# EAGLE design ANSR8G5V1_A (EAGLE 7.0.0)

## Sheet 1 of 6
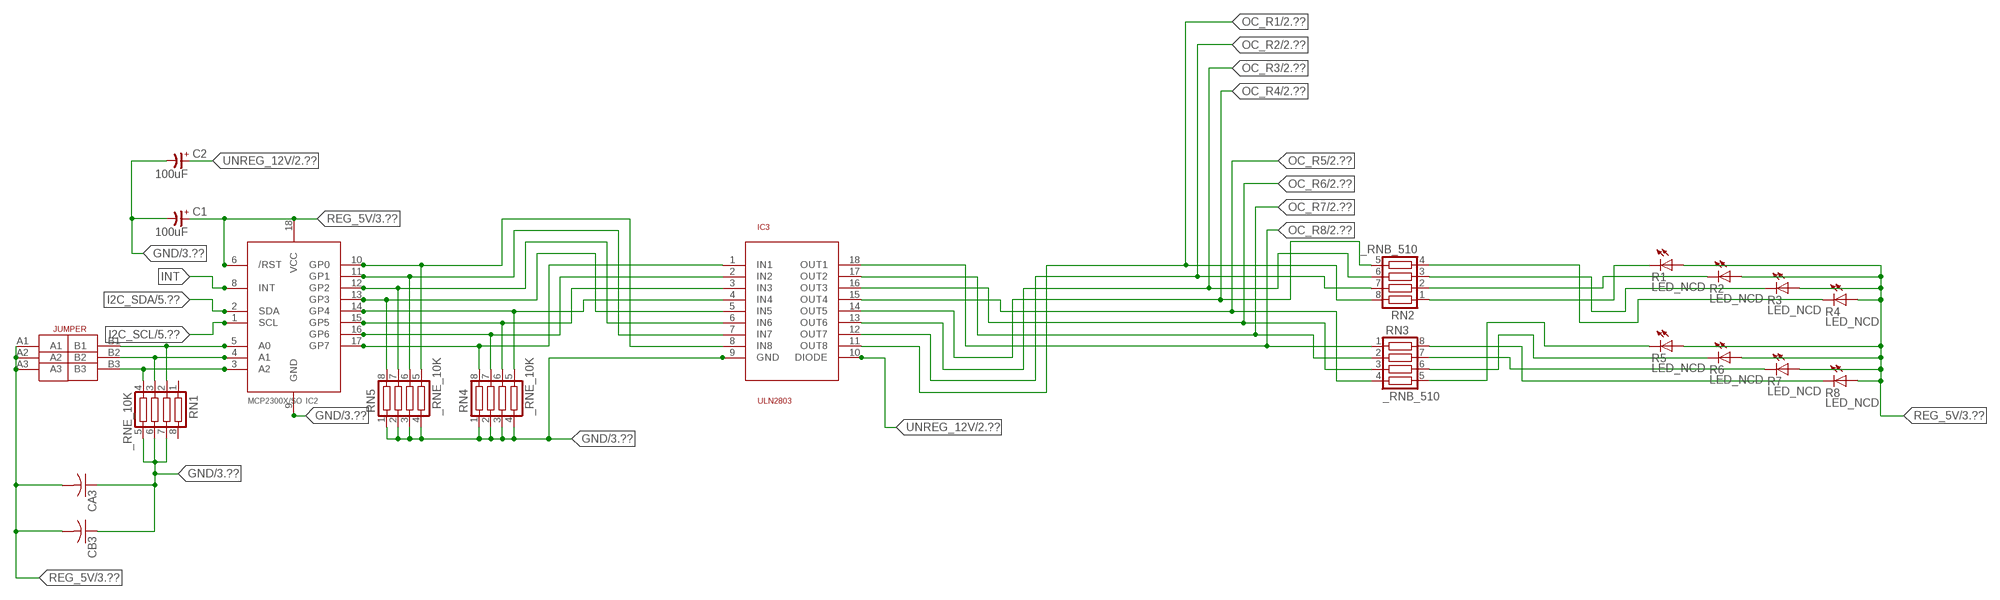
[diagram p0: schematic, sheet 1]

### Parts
C1  100uF  CP-E-025X060  [E-025X060]
C2  100uF  CP-E-025X060  [E-025X060]
CA3  CC1206KRX7R9BB104C1206K  [CC1206KRX7R9BB104]
CB3  TMK316F106ZL-TC1206K  [TMK316F106ZL-T]
IC2  MCP2300X/SO  [SO18W]
IC3  ULN2803  [SO18L]
R1  LED_NCD  [CHIPLED_0603]
R2  LED_NCD  [CHIPLED_0603]
R3  LED_NCD  [CHIPLED_0603]
R4  LED_NCD  [CHIPLED_0603]
R5  LED_NCD  [CHIPLED_0603]
R6  LED_NCD  [CHIPLED_0603]
R7  LED_NCD  [CHIPLED_0603]
R8  LED_NCD  [CHIPLED_0603]
RN1  _RNE_10K  [RNE]
RN2  _RNB_510  [RNB]
RN3  _RNB_510  [RNB]
RN4  _RNE_10K  [RNE]
RN5  _RNE_10K  [RNE]
U$18  JUMPER_3X2  [JUMPER_3X2]

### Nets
GND: C1.- C2.- CA3.1 CB3.1 IC2.9(GND) IC3.9(GND) RN1.5 RN1.6 RN1.7 RN4.1 RN4.2 RN4.3 RN4.4 RN5.1 RN5.2 RN5.3 RN5.4 ; also sheet 3,4,5,6
GP4: IC2.14(GP4) IC3.4(IN4) RN4.5
GP6: IC2.16(GP6) IC3.2(IN2) RN4.7
I2C_SCL: IC2.1(SCL) ; also sheet 5,6
I2C_SDA: IC2.2(SDA) ; also sheet 5,6
INT: IC2.8(INT)
N$6: IC2.5(A0) RN1.2 U$18.B1
N$7: IC2.4(A1) RN1.3 U$18.B2
N$8: IC2.3(A2) RN1.4 U$18.B3
N$20: R1.C RN2.1
N$21: IC2.12(GP2) IC3.6(IN6) RN5.7
N$22: IC2.11(GP1) IC3.7(IN7) RN5.6
N$23: IC2.10(GP0) IC3.8(IN8) RN5.5
N$29: R2.C RN2.2
N$30: R3.C RN2.3
N$31: R4.C RN2.4
N$32: R8.C RN3.8
N$81: R7.C RN3.7
N$82: R6.C RN3.6
N$83: R5.C RN3.5
N$89: IC2.13(GP3) IC3.5(IN5) RN5.8
N$93: IC2.15(GP5) IC3.3(IN3) RN4.6
N$94: IC2.17(GP7) IC3.1(IN1) RN4.8
OC_R1: IC3.11(OUT8) RN2.8 ; also sheet 2
OC_R2: IC3.12(OUT7) RN2.7 ; also sheet 2
OC_R3: IC3.13(OUT6) RN2.6 ; also sheet 2
OC_R4: IC3.14(OUT5) RN2.5 ; also sheet 2
OC_R5: IC3.15(OUT4) RN3.4 ; also sheet 2
OC_R6: IC3.16(OUT3) RN3.3 ; also sheet 2
OC_R7: IC3.17(OUT2) RN3.2 ; also sheet 2
OC_R8: IC3.18(OUT1) RN3.1 ; also sheet 2
REG_5V: C1.+ CA3.2 CB3.2 IC2.6(/RST) IC2.18(VCC) R1.A R2.A R3.A R4.A R5.A R6.A R7.A R8.A U$18.A1 U$18.A2 U$18.A3 ; also sheet 3,4,5,6
UNREG_12V: C2.+ IC3.10(DIODE) ; also sheet 2,3
Unconnected: RN1.1 RN1.8

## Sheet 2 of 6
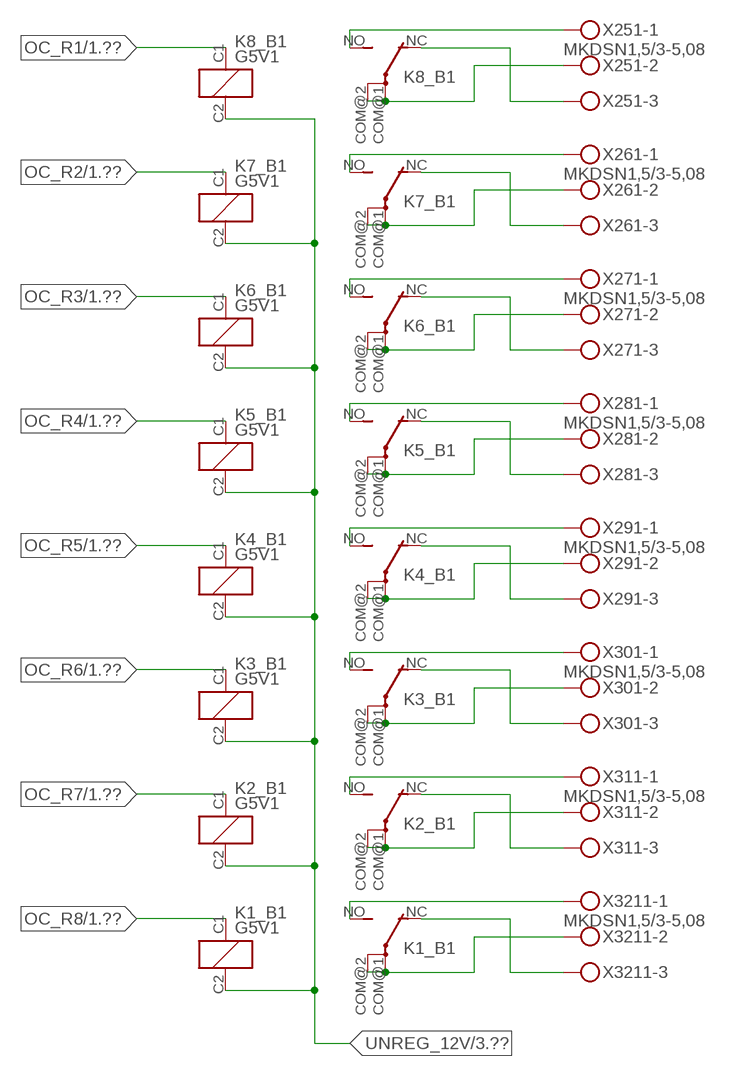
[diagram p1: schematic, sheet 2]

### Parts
K1_B1  G5V1  [G5V1]
K2_B1  G5V1  [G5V1]
K3_B1  G5V1  [G5V1]
K4_B1  G5V1  [G5V1]
K5_B1  G5V1  [G5V1]
K6_B1  G5V1  [G5V1]
K7_B1  G5V1  [G5V1]
K8_B1  G5V1  [G5V1]
X251  MKDSN1,5/3-5,08  [MKDSN1,5/3-5,08]
X261  MKDSN1,5/3-5,08  [MKDSN1,5/3-5,08]
X271  MKDSN1,5/3-5,08  [MKDSN1,5/3-5,08]
X281  MKDSN1,5/3-5,08  [MKDSN1,5/3-5,08]
X291  MKDSN1,5/3-5,08  [MKDSN1,5/3-5,08]
X301  MKDSN1,5/3-5,08  [MKDSN1,5/3-5,08]
X311  MKDSN1,5/3-5,08  [MKDSN1,5/3-5,08]
X3211  MKDSN1,5/3-5,08  [MKDSN1,5/3-5,08]

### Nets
N$203: K8_B1.COM@1(2:P) K8_B1.COM@2(2:P) X251.2
N$204: K8_B1.NC(2:O) X251.3
N$205: K8_B1.NO(2:S) X251.1
N$206: K7_B1.NO(2:S) X261.1
N$207: K6_B1.NO(2:S) X271.1
N$208: K7_B1.NC(2:O) X261.3
N$209: K7_B1.COM@1(2:P) K7_B1.COM@2(2:P) X261.2
N$210: K6_B1.NC(2:O) X271.3
N$211: K6_B1.COM@1(2:P) K6_B1.COM@2(2:P) X271.2
N$212: K5_B1.NC(2:O) X281.3
N$213: K5_B1.COM@1(2:P) K5_B1.COM@2(2:P) X281.2
N$214: K5_B1.NO(2:S) X281.1
N$215: K4_B1.NO(2:S) X291.1
N$216: K4_B1.NC(2:O) X291.3
N$217: K4_B1.COM@1(2:P) K4_B1.COM@2(2:P) X291.2
N$218: K3_B1.NO(2:S) X301.1
N$219: K3_B1.NC(2:O) X301.3
N$220: K3_B1.COM@1(2:P) K3_B1.COM@2(2:P) X301.2
N$221: K2_B1.NO(2:S) X311.1
N$222: K2_B1.NC(2:O) X311.3
N$223: K2_B1.COM@1(2:P) K2_B1.COM@2(2:P) X311.2
N$224: K1_B1.NO(2:S) X3211.1
N$225: K1_B1.NC(2:O) X3211.3
N$226: K1_B1.COM@1(2:P) K1_B1.COM@2(2:P) X3211.2
OC_R1: K8_B1.C1(1:C1) ; also sheet 1
OC_R2: K7_B1.C1(1:C1) ; also sheet 1
OC_R3: K6_B1.C1(1:C1) ; also sheet 1
OC_R4: K5_B1.C1(1:C1) ; also sheet 1
OC_R5: K4_B1.C1(1:C1) ; also sheet 1
OC_R6: K3_B1.C1(1:C1) ; also sheet 1
OC_R7: K2_B1.C1(1:C1) ; also sheet 1
OC_R8: K1_B1.C1(1:C1) ; also sheet 1
UNREG_12V: K1_B1.C2(1:C2) K2_B1.C2(1:C2) K3_B1.C2(1:C2) K4_B1.C2(1:C2) K5_B1.C2(1:C2) K6_B1.C2(1:C2) K7_B1.C2(1:C2) K8_B1.C2(1:C2) ; also sheet 1,3

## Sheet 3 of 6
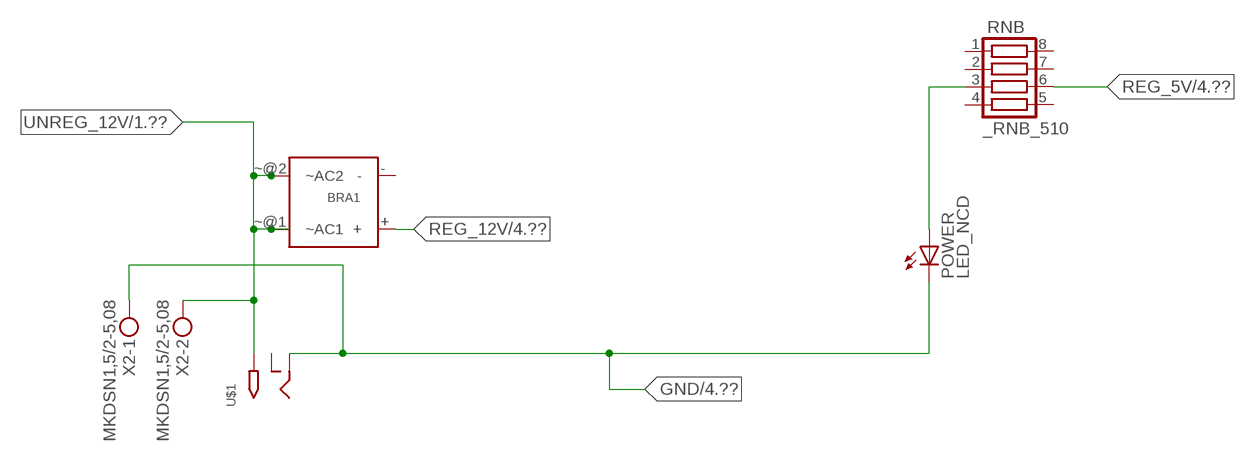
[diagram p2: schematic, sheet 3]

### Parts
BRA1  MB2S_  [MB2S]
POWER  LED_NCD  [CHIPLED_0603]
RNB  _RNB_510  [RNB]
U$1  2.1MMJACK  [PJ-102A]
X2  MKDSN1,5/2-5,08  [MKDSN1,5/2-5,08]

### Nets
GND: POWER.C U$1.RING X2.1 ; also sheet 1,4,5,6
N$2: POWER.A RNB.3
REG_5V: RNB.6 ; also sheet 1,4,5,6
REG_12V: BRA1.+ ; also sheet 4
UNREG_12V: BRA1.~@1(~AC1) BRA1.~@2(~AC2) U$1.TIP X2.2 ; also sheet 1,2
Unconnected: BRA1.- RNB.1 RNB.2 RNB.4 RNB.5 RNB.7 RNB.8 U$1.RING_SW

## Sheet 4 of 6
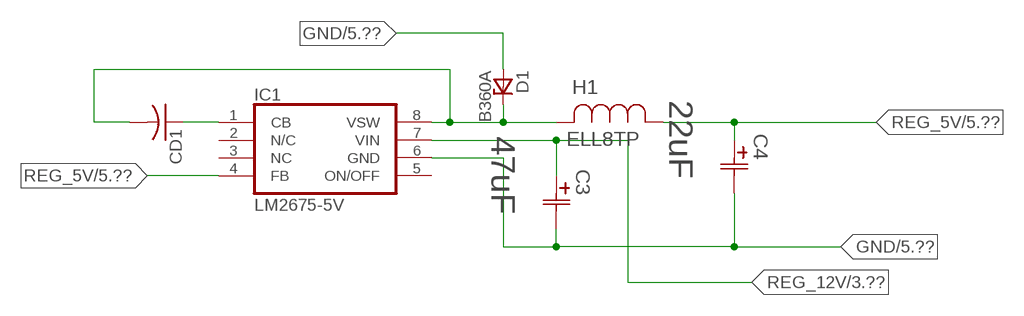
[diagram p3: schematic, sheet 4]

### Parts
C3  47uF  490-5463-6-NDCAP  [C2917(7343)-Y]
C4  22uF  490-5463-6-NDCAP  [C2917(7343)-Y]
CD1  _CD_10NF_50VC1206K  [_CD_10NF_50V]
D1  B360A  [DO214AC_ZENER]
H1  ELL8TP  [IND_ELL8TP]
IC1  LM2675-5V  LM2675  [SO-8]

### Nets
GND: C3.2(C2) C4.2(C2) D1.A IC1.6(GND) ; also sheet 1,3,5,6
N$1: CD1.2 D1.C H1.2 IC1.8(VSW)
N$3: CD1.1 IC1.1(CB)
REG_5V: C4.1(C1) H1.1 IC1.4(FB) ; also sheet 1,3,5,6
REG_12V: C3.1(C1) IC1.7(VIN) ; also sheet 3
Unconnected: IC1.2(N/C) IC1.5(ON/OFF)

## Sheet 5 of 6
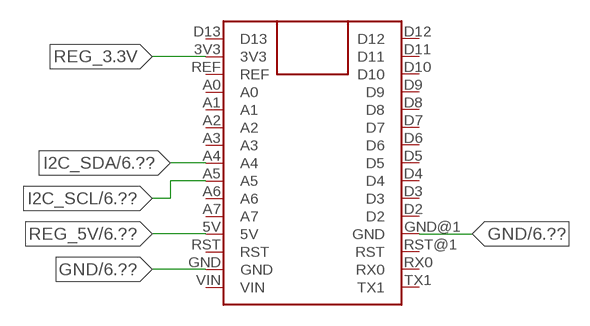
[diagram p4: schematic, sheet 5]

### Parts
FOR_NANO  ARDUINO_NANO  [ARDUINO_NANO]

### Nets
GND: FOR_NANO.GND FOR_NANO.GND@1(GND) ; also sheet 1,3,4,6
I2C_SCL: FOR_NANO.A5 ; also sheet 1,6
I2C_SDA: FOR_NANO.A4 ; also sheet 1,6
REG_3.3V: FOR_NANO.3V3
REG_5V: FOR_NANO.5V ; also sheet 1,3,4,6
Unconnected: FOR_NANO.A0 FOR_NANO.A1 FOR_NANO.A2 FOR_NANO.A3 FOR_NANO.A6 FOR_NANO.A7 FOR_NANO.D2 FOR_NANO.D3 FOR_NANO.D4 FOR_NANO.D5 FOR_NANO.D6 FOR_NANO.D7 FOR_NANO.D8 FOR_NANO.D9 FOR_NANO.D10 FOR_NANO.D11 FOR_NANO.D12 FOR_NANO.D13 FOR_NANO.REF FOR_NANO.RST FOR_NANO.RST@1(RST) FOR_NANO.RX0 FOR_NANO.TX1 FOR_NANO.VIN

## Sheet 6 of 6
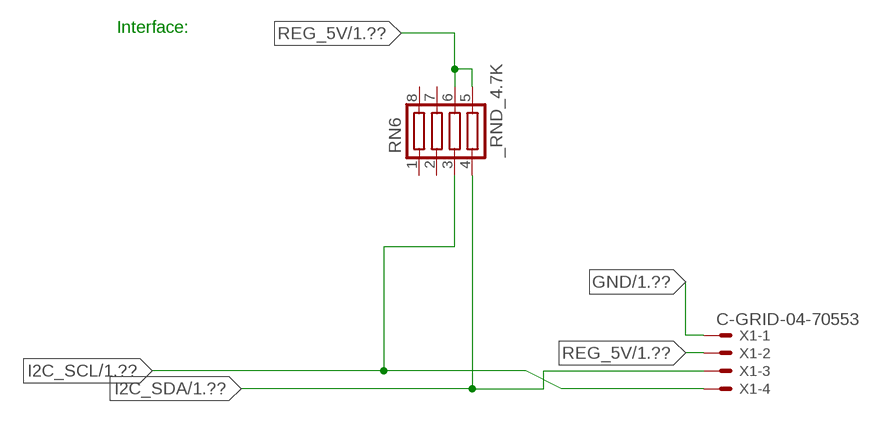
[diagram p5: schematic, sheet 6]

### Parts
RN6  _RND_4.7K  [RND]
X1  C-GRID-04-70553  [70553-04]

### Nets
GND: X1.1 ; also sheet 1,3,4,5
I2C_SCL: RN6.3 X1.4 ; also sheet 1,5
I2C_SDA: RN6.4 X1.3 ; also sheet 1,5
REG_5V: RN6.5 RN6.6 X1.2 ; also sheet 1,3,4,5
Unconnected: RN6.1 RN6.2 RN6.7 RN6.8

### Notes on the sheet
- Interface:

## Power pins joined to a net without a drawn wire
NC: IC1.3(NC)

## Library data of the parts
BRA1 = NCD_ULTIMATE_LIBRARY:MB2S: Bridge Rectifier BRA MB2S 200V 500ma Digikey MB2S-TPMSTR-ND/MB2S-TP
C1 C2 = NCD_ULTIMATE_LIBRARY:CP-: Capacitors All Kinds POLARIZED CAP
C3 C4 = NCD_ULTIMATE_bhaskar:490-5463-6-ND: NCD CAP
CA3 = NCD_ULTIMATE_LIBRARY:CC1206KRX7R9BB104: Capacitor CA .1uF 50V SMT C1206K CC1206KRX7R9BB104
CB3 = NCD_ULTIMATE_LIBRARY:TMK316F106ZL-T: Capacitor CB 10uF SMT 1206 TMK316F106ZL-T
CD1 = NCD_ULTIMATE_LIBRARY:_CD_10NF_50V: Capacitor 10nF SMT
D1 = NCD_ULTIMATE_bhaskar:B360A: NCD DIODE B350A/B360A
FOR_NANO = NCD_ULTIMATE_CONNECTORS:ARDUINO_NANO
H1 = NCD_ULTIMATE_bhaskar:ELL8TP: NCD coil
IC1 = NCD_ULTIMATE_bhaskar:LM2675: LM2675 NCD http://www.ti.com/lit/ds/symlink/lm2675.pdf
IC2 = NCD_ULTIMATE_LIBRARY:MCP2300X: Semiconductor Port Expander I/O 8-Bit I2C MCP23008 Inexpensive i2c i/o expander - 8 general purpose i/o pins with optional pullups
IC3 = NCD_ULTIMATE_LIBRARY:ULN2803: Semiconductor 8 O.C. N-Channel Transistor Driver Digikey ULN2803AFWGCELTR-ND/ULN2803AFWG,C,EL
K1_B1 K2_B1 K3_B1 K4_B1 K5_B1 K6_B1 K7_B1 K8_B1 = NCD_ULTIMATE_LIBRARY:G5V1: RELAY 1 x switch, 0.5 A/125 V AC, 1 A/24 V DC , Omron
POWER = NCD_ULTIMATE_bhaskar:LED_NCD
R1-R8 = NCD_ULTIMATE_LIBRARY:LED_NCD: LED Digikey 754-1132-2-ND/APT2012SRCPRV
RN1 RN4 RN5 = NCD_ULTIMATE_LIBRARY:_RNE_10K: Resistor Array RNE SMT 10K x 4 Single Resistor Source: http://www.ctscorp.com/components/Datasheets/CTSChipArrayDs.pdf Digikey 742C083103JPTR-ND/742C083103JP; OC_FARNELL: unknown; OC_NEWARK: unknown
RN2 RN3 RNB = NCD_ULTIMATE_LIBRARY:_RNB_510: Resistor Array RNB SMT 510 x 4 Single Resistor Source: http://www.ctscorp.com/components/Datasheets/CTSChipArrayDs.pdf Digikey 742C083511JPTR-ND/ 742C083511JP; OC_FARNELL: unknown; OC_NEWARK: unknown
RN6 = NCD_ULTIMATE_LIBRARY:_RND_4.7K: Resistor Array RND SMT 4.7K x 4 Single Resistor Source: http://www.ctscorp.com/components/Datasheets/CTSChipArrayDs.pdf Digikey 742C083472JPTR-ND/742C083472JP; OC_FARNELL: unknown; OC_NEWARK: unknown
U$1 = NCD_ULTIMATE_CONNECTORS:2.1MMJACK: 2.1mm x 5.5mm DC jack with internal switch. Digikey part #PJ-102A, 4UCON part #05537 By microbuilder.eu
U$18 = NCD_ULTIMATE_CONNECTORS:JUMPER_3X2
X1 = NCD_ULTIMATE_CONNECTORS:C-GRID-04: CONNECTOR 4-Pos I2C wire to board 2.54 mm (0.100") pitch header Digikey WM1342-ND/0015912045; OC_FARNELL: unknown; OC_NEWARK: unknown
X2 = NCD_ULTIMATE_CONNECTORS:MKDSN1,5/2-5,08: MKDSN 1,5/ 2-5,08 Printklemme
X251 X261 X271 X281 X291 X301 X311 X3211 = NCD_ULTIMATE_CONNECTORS:MKDSN1,5/3-5,08: MKDSN 1,5/ 3-5,08 Printklemme Nennstrom: 13,5 A Nennspannung: 250 V Rastermaß: 5,08 mm Polzahl: 3 Anschlussart: Schraubanschluss Montage: Löten Anschlussrichtung Leiter/Platine: 0 ° Artikelnummer: 1729131 Source: http://eshop.phoenixcontact.com .. 1729131.pdf

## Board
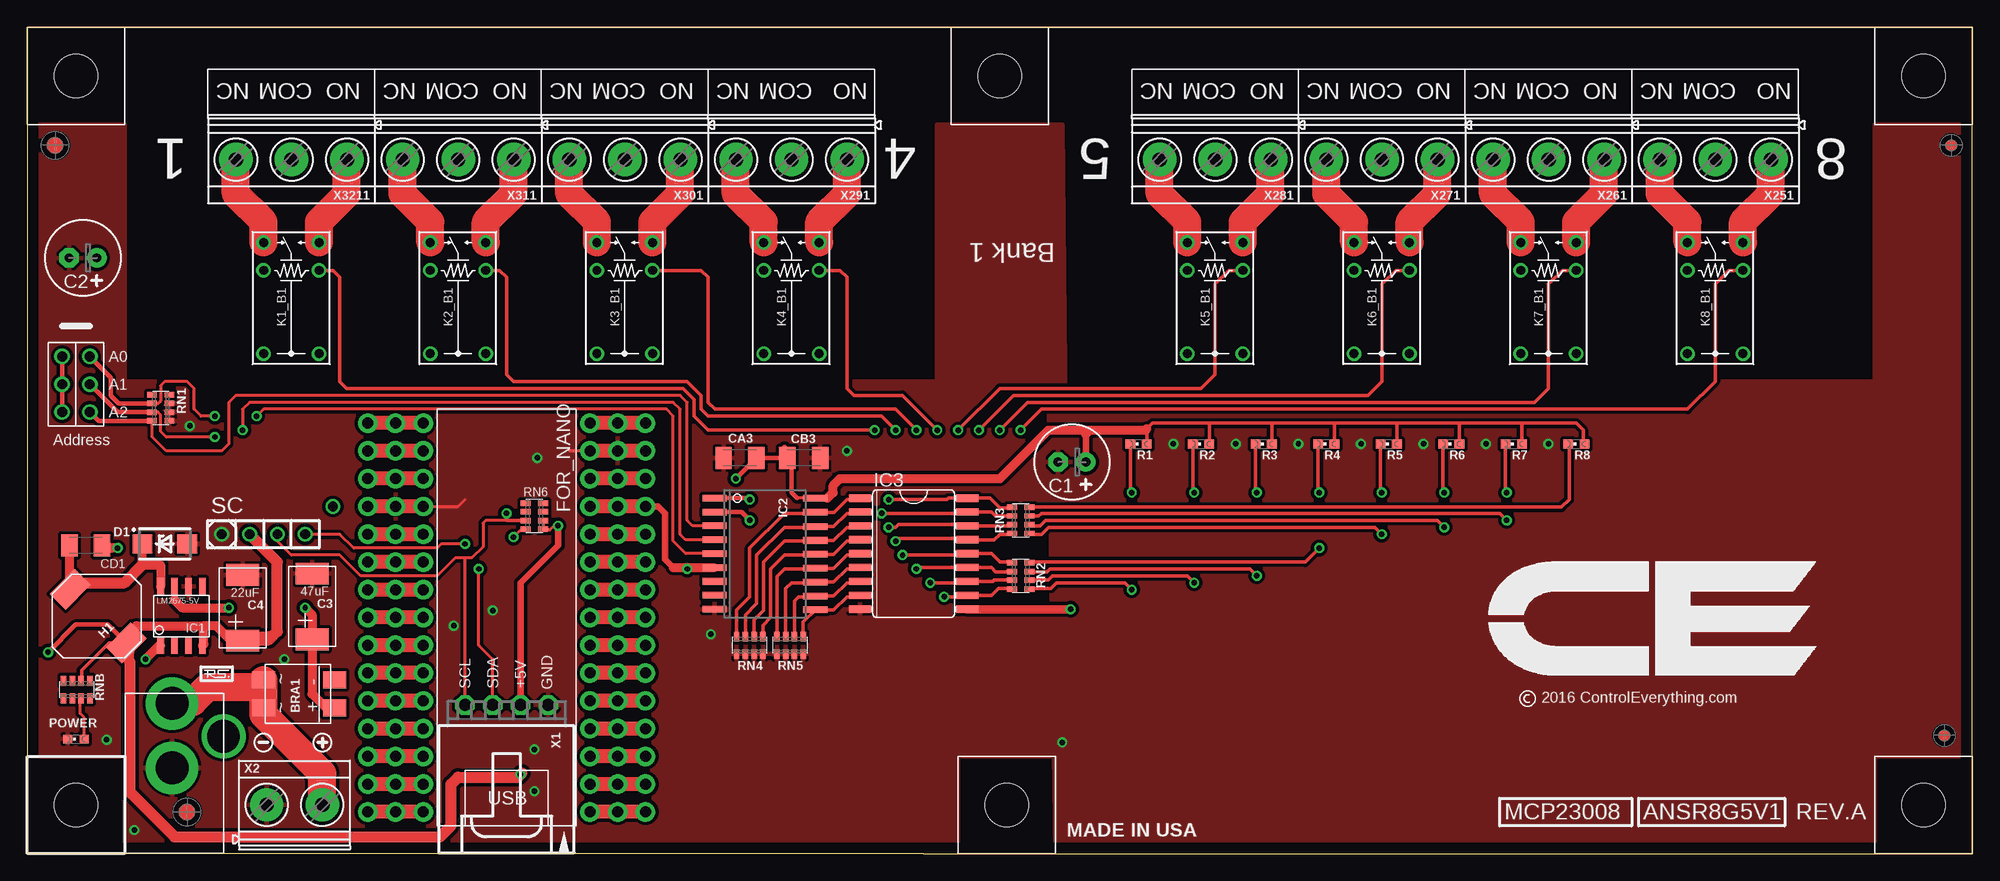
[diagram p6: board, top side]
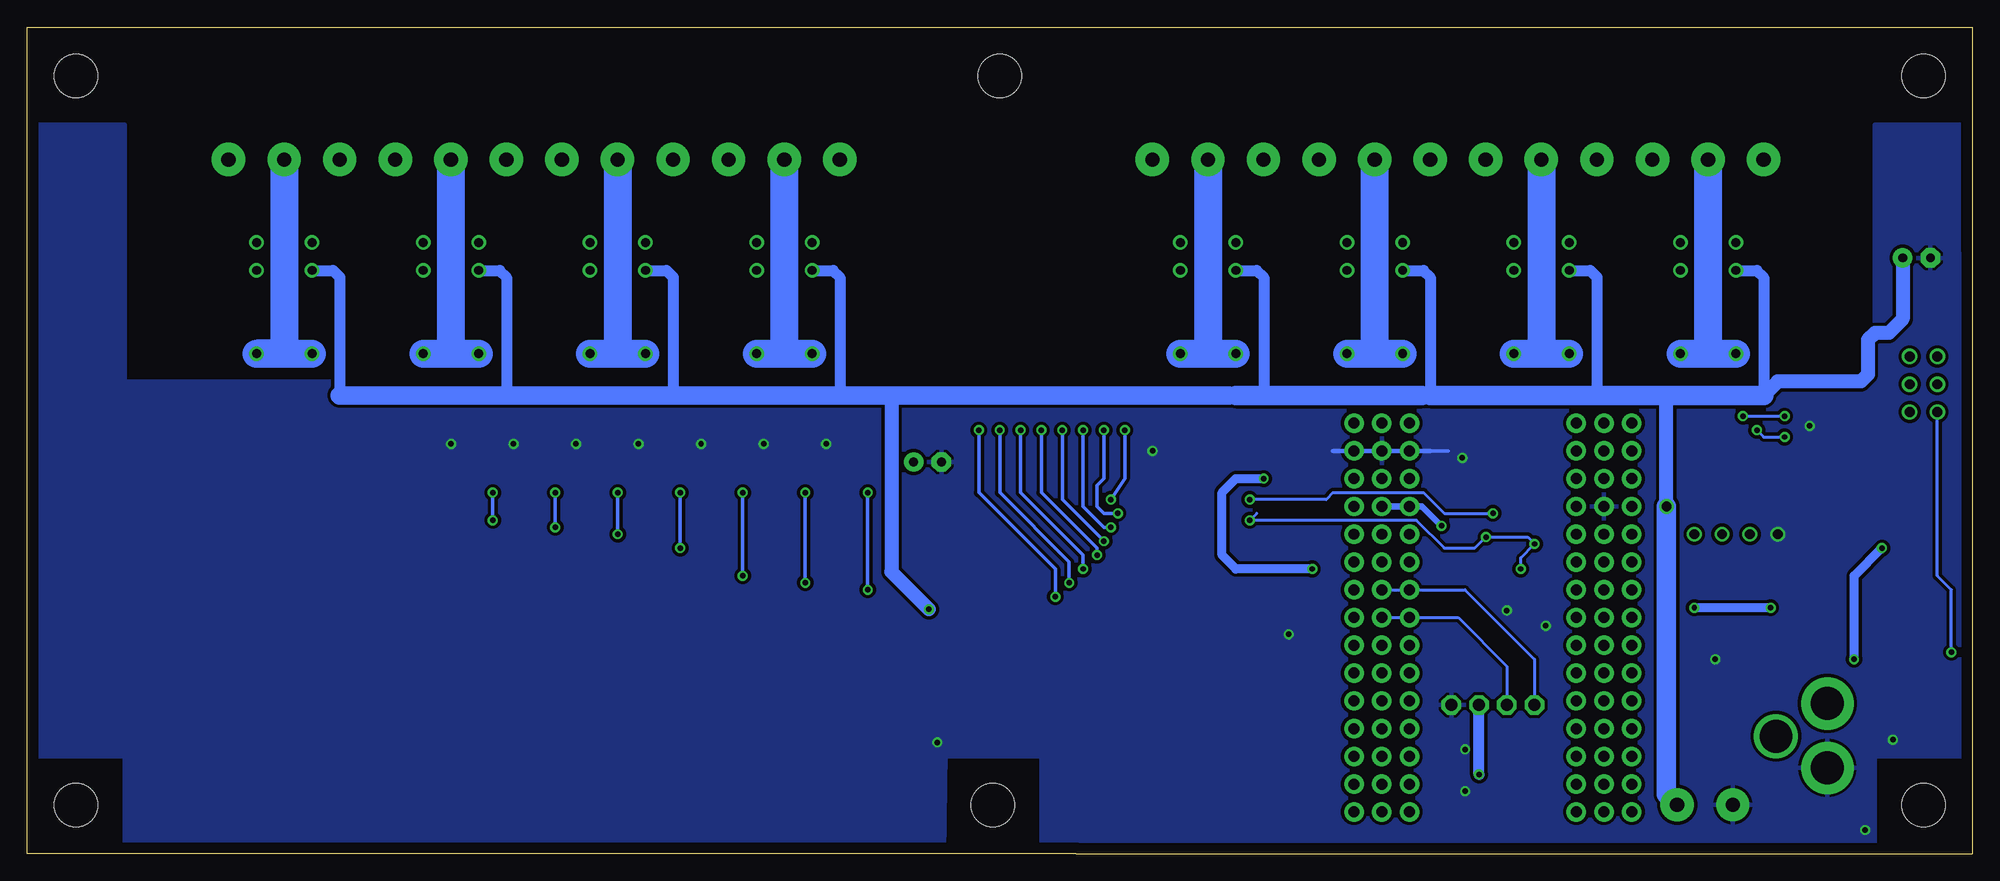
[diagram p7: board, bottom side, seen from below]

Size 177.8 x 75.56 mm. Coordinates in mm from the lower left corner, seen from the top.
Outline: 81.92,0 83.17,0
Outline: 0,56.19 0,55.24
Outline: 0,55.24 0,0 81.92,0
Outline: 81.92,0 177.8,0 177.8,75.56 0,75.56 0,55.24
Copper layers (1*16): Top 0.035mm / dielectric 1.5mm / Bottom 0.035mm
Design rules "default": minimum track width 10mil, minimum drill 24mil, track to track 8mil, track to pad 8mil, pad to pad 8mil, via to via 8mil, smd to smd 8mil, copper to edge 40mil, drill to drill 8mil, minimum pad ring 10mil, minimum via ring 8mil, stop-mask expansion 4mil, vias tented up to drill 0mil, thermal gap 10mil
Holes 3.96 mm at 4.45,4.45 4.45,4.45 4.45,4.45

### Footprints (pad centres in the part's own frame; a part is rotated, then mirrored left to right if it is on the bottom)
MB2S = smd 1.55 x 2.1: + 0,-6.5; - 2.54,-6.5; ~@1 0,0; ~@2 2.54,0
E-025X060 = drill 0.813 pad 1.778: + -1.27,0 | drill 0.813 pad 1.778 octagon: - 1.27,0
C2917(7343)-Y = smd 2 x 3: 1 -3,0; 2 3,0
CC1206KRX7R9BB104 = smd 1.5 x 2: 1 -1.5,0; 2 1.5,0
TMK316F106ZL-T = smd 1.5 x 2: 1 -1.5,0; 2 1.5,0
_CD_10NF_50V = smd 1.5 x 2: 1 -1.5,0; 2 1.5,0
DO214AC_ZENER = smd 1.8 x 1.7: A 2.05,0; C -2.05,0
ARDUINO_NANO = drill 1 pad 1.778: 3V1 -2.54,-2.54; 3V3 0,-2.54; 5V 0,-27.94; 5V1 -2.54,-27.94; A0 0,-7.62; A1 0,-10.16; A2 0,-12.7; A3 0,-15.24; A4 0,-17.78; A5 0,-20.32; A6 0,-22.86; A7 0,-25.4; A8 -2.54,-7.62; A9 -2.54,-10.16; A10 -2.54,-12.7; A11 -2.54,-15.24; A12 -2.54,-17.78; A13 -2.54,-20.32; A14 -2.54,-22.86; A15 -2.54,-25.4; D1 -2.54,0; D2 20.32,-25.4; D3 20.32,-22.86; D4 20.32,-20.32; D5 20.32,-17.78; D6 20.32,-15.24; D7 20.32,-12.7; D8 20.32,-10.16; D9 20.32,-7.62; D10 20.32,-5.08; D11 20.32,-2.54; D12 20.32,0; D13 0,0; D14 22.86,0; D15 22.86,-2.54; D16 22.86,-5.08; D17 22.86,-7.62; D18 22.86,-10.16; D19 22.86,-12.7; D20 22.86,-15.24; D21 22.86,-17.78; D22 22.86,-20.32; D23 22.86,-22.86; D24 22.86,-25.4; GND 0,-33.02; GND1 -2.54,-33.02; GND@1 20.32,-27.94; GND@2 22.86,-27.94; P$16 2.54,0; P$17 2.54,-2.54; P$18 2.54,-5.08; P$19 2.54,-7.62; P$20 2.54,-10.16; P$21 2.54,-12.7; P$22 2.54,-15.24; P$23 2.54,-17.78; P$24 2.54,-20.32; P$25 2.54,-22.86; P$26 2.54,-25.4; P$27 2.54,-27.94; P$28 2.54,-30.48; P$29 2.54,-33.02; P$30 2.54,-35.56; P$31 17.78,0; P$32 17.78,-2.54; P$33 17.78,-5.08; P$34 17.78,-7.62; P$35 17.78,-10.16; P$36 17.78,-12.7; P$37 17.78,-15.24; P$38 17.78,-17.78; P$39 17.78,-20.32; P$40 17.78,-22.86; P$41 17.78,-25.4; P$42 17.78,-27.94; P$43 17.78,-30.48; P$44 17.78,-33.02; P$45 17.78,-35.56; REF 0,-5.08; REF1 -2.54,-5.08; RST 0,-30.48; RST1 -2.54,-30.48; RST@1 20.32,-30.48; RST@2 22.86,-30.48; RX0 20.32,-33.02; RX1 22.86,-33.02; TX1 20.32,-35.56; TX2 22.86,-35.56; VIN 0,-35.56; VIN1 -2.54,-35.56
IND_ELL8TP = smd 2.054 x 3.2 rotated 45: 1 -2.442,-2.696; 2 2.442,2.442
SO-8 = smd 0.6 x 1.55: 1 -1.905,-2.69; 2 -0.635,-2.69; 3 0.635,-2.69; 4 1.905,-2.69; 5 1.905,2.71; 6 0.635,2.71; 7 -0.635,2.71; 8 -1.905,2.71
SO18W = smd 0.6 x 2.2: 1 -4.445,-4.6; 2 -3.175,-4.6; 3 -1.905,-4.6; 4 -0.635,-4.6; 5 0.635,-4.6; 6 1.905,-4.6; 7 3.175,-4.6; 8 4.445,-4.6; 9 5.715,-4.6; 10 5.775,4.6; 11 4.505,4.6; 12 3.235,4.6; 13 1.965,4.6; 14 0.695,4.6; 15 -0.575,4.6; 16 -1.845,4.6; 17 -3.145,4.6; 18 -4.445,4.6
SO18L = smd 0.66 x 2.032: 1 -5.08,-4.902; 2 -3.81,-4.902; 3 -2.54,-4.902; 4 -1.27,-4.902; 5 0,-4.902; 6 1.27,-4.902; 7 2.54,-4.902; 8 3.81,-4.902; 9 5.08,-4.902; 10 5.08,4.902; 11 3.81,4.902; 12 2.54,4.902; 13 1.27,4.902; 14 0,4.902; 15 -1.27,4.902; 16 -2.54,4.902; 17 -3.81,4.902; 18 -5.08,4.902
G5V1 = drill 0.813: C1 -2.54,2.54; C2 -2.54,-2.54; COM@1 5.08,-2.54; COM@2 5.08,2.54; NC -5.08,-2.54; NO -5.08,2.54
CHIPLED_0603 = smd 0.8 x 0.8: A 0,-0.75; C 0,0.75
CHIPLED_0603' = smd 0.8 x 0.876: A 0,-0.75; C 0,0.75
RNE = smd 0.5 x 0.9: 1 -1.2,-0.8; 2 -0.4,-0.8; 3 0.4,-0.8; 4 1.2,-0.8; 5 1.2,0.8; 6 0.4,0.8; 7 -0.4,0.8; 8 -1.2,0.8
RNB = smd 0.5 x 0.9: 1 -1.2,-0.8; 2 -0.4,-0.8; 3 0.4,-0.8; 4 1.2,-0.8; 5 1.2,0.8; 6 0.4,0.8; 7 -0.4,0.8; 8 -1.2,0.8
RND = smd 0.5 x 0.9: 1 -1.2,-0.8; 2 -0.4,-0.8; 3 0.4,-0.8; 4 1.2,-0.8; 5 1.2,0.8; 6 0.4,0.8; 7 -0.4,0.8; 8 -1.2,0.8
PJ-102A = drill 3 pad 4.8: RING 0.1,-3.39; TIP 0.1,-9.29 | drill 3 pad 3.251: RING_SW -4.6,-6.29
PCB_MOUNTING_HOLE = hole 3.962: 4.445,4.445
JUMPER_3X2 = drill 0.9: A1 0,5.08; A2 0,2.54; A3 0,0; B1 2.54,5.08; B2 2.54,2.54; B3 2.54,0
70553-04 = drill 1.1 pad 1.778 octagon: 1 -3.81,-7.62; 2 -1.27,-7.62; 3 1.27,-7.62; 4 3.81,-7.62
MKDSN1,5/2-5,08 = drill 1.3 pad 3.048: 1 -2.561,0.025; 2 2.519,0.025
MKDSN1,5/3-5,08 = drill 1.3 pad 3.048: 1 -7.641,0.025; 2 -2.561,0.025; 3 2.519,0.025

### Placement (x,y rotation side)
BRA1  21.59,13.34 90 top
C1  95.5,35.81 180 top
C2  5.08,54.48 180 top
C3  26.04,22.61 90 top
C4  19.68,22.48 90 top
CA3  65.15,36.2 0 top
CB3  70.99,36.2 180 top
CD1  5.33,28.19 180 top
D1  12.57,28.32 0 top
FOR_NANO  53.98,3.81 180 top
H1  6.35,21.72 90 top
IC1  14.1,21.72 0 top
IC2  67.44,28.07 270 top
IC3  81.03,27.43 270 top
K1_B1  24.13,50.8 270 top
K2_B1  39.37,50.8 270 top
K3_B1  54.61,50.8 270 top
K4_B1  69.85,50.8 270 top
K5_B1  108.58,50.8 270 top
K6_B1  123.83,50.8 270 top
K7_B1  139.06,50.8 270 top
K8_B1  154.31,50.8 270 top
POWER  4.45,10.48 90 top
R1  LED_NCD  [CHIPLED_0603']  101.6,37.47 90 top
R2  LED_NCD  [CHIPLED_0603']  107.31,37.47 90 top
R3  LED_NCD  [CHIPLED_0603']  113.03,37.47 90 top
R4  LED_NCD  [CHIPLED_0603']  118.75,37.47 90 top
R5  LED_NCD  [CHIPLED_0603']  124.46,37.47 90 top
R6  LED_NCD  [CHIPLED_0603']  130.18,37.47 90 top
R7  LED_NCD  [CHIPLED_0603']  135.89,37.47 90 top
R8  LED_NCD  [CHIPLED_0603']  141.6,37.47 90 top
RN1  12.19,40.77 270 top
RN2  90.81,25.4 90 top
RN3  90.81,30.48 270 top
RN4  66.04,19.05 0 top
RN5  69.72,19.05 0 top
RN6  46.35,30.86 270 top
RNB  4.51,14.99 0 top
U$1  13.34,4.45 180 top
U$2  [VISION_REF15]  14.61,3.81 0 top
U$3  [ICON_MINUS]  21.59,10.16 180 top
U$4  [VISION_REF10]  175.26,10.79 270 top
U$5  PCB_MOUNTING_HOLE  [PCB_MOUNTING_HOLE]  177.8,66.67 90 top
U$6  PCB_MOUNTING_HOLE  [PCB_MOUNTING_HOLE]  93.98,0 90 top
U$7  PCB_MOUNTING_HOLE  [PCB_MOUNTING_HOLE]  93.34,66.67 90 top
U$8  PCB_MOUNTING_HOLE  [PCB_MOUNTING_HOLE]  8.89,66.67 90 top
U$9  [ICON_PLUS]  26.99,10.16 90 top
U$11  PCB_MOUNTING_HOLE  [PCB_MOUNTING_HOLE]  177.8,0 90 top
U$12  PCB_MOUNTING_HOLE  [PCB_MOUNTING_HOLE]  177.8,66.67 90 top
U$15  [VISION_REF15]  2.54,64.77 270 top
U$18  3.17,40.39 0 top
U$21  [ICON_USA]  95,1.52 0 top
U$28  [VISION_REF10]  175.9,64.77 270 top
X1  43.81,5.97 180 top
X2  24.45,4.45 0 top
X251  151.76,63.5 180 top
X261  136.53,63.5 180 top
X271  121.28,63.5 180 top
X281  106.05,63.5 180 top
X291  67.31,63.5 180 top
X301  52.07,63.5 180 top
X311  36.83,63.5 180 top
X3211  21.59,63.5 180 top

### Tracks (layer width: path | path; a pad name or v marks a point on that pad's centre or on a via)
GND  (via drill 0.5, 0.9)
  Top 0.254: 36.2,31.75 39.37,31.75 40.01,32.39 | FOR_NANO.GND@1 32.38,31.75 | 56.52,36.83 49.53,36.83
  Top 1.016: X1.1 47.62,13.74
  Bottom 0.254: 51.44,36.83 FOR_NANO.GND
  Bottom 0.305: 47.88,36.83 49.53,36.83 51.44,36.83
  Bottom 0.406: 49.53,36.83 58.42,36.83
  other vias: 14.86,39.12 62.48,20.07 127.64,37.47 94.61,10.16 133.35,37.47 139.06,37.47 121.92,37.47 116.2,37.47 110.49,37.47 104.78,37.47 74.93,36.83 9.78,2.16 17.78,29.21 46.35,9.53 46.61,36.2 46.35,5.72 42.55,22.23 38.99,20.83 7.24,10.41 23.5,17.78
  pour Bottom (isolate 0.305): -1.91,8.89 8.89,8.89 8.89,0 85.09,0 85.09,8.89 95.25,8.89 94.61,66.67 83.19,66.67 83.19,43.18 8.89,43.18 8.89,66.67 -1.91,66.67
  pour Top (isolate 0.305): -3.81,8.89 8.89,8.89 8.89,0 85.09,0 85.09,8.89 95.25,8.89 94.61,66.67 83.19,66.67 83.19,43.18 8.89,43.18 8.89,66.67 -3.81,66.67
  pour Top (isolate 0.305): 93.34,43.18 168.91,43.18 168.91,66.67 179.71,66.67 179.71,8.89 168.91,8.89 168.91,0 93.98,0
  pour Bottom (isolate 0.305): 93.98,0 93.34,43.18 168.91,43.18 168.91,66.67 182.25,66.67 182.25,8.89 168.91,8.89 168.91,0
GP4
  Top 0.305: RN4.5 67.24,20.88 67.94,21.59 67.94,26.04 69.22,27.3 71.97,27.3 IC2.14 73.73,27.37 74.93,28.57 76,28.57 IC3.4
GP6
  Top 0.305: RN4.7 65.64,21.83 66.67,22.86 66.67,27.3 69.22,29.84 71.97,29.84 IC2.16 73.73,29.91 74.93,31.12 76,31.12 IC3.2
I2C_SCL  (via drill 0.5, 0.9)
  Top 0.254: 40.01,27.05 40.64,27.05 41.66,28.07 41.66,30.23 41.89,30.46 RN6.3 45.54,30.48 43.81,30.48 v43.81,31.12 | 40.01,27.05 39.12,27.05 37.47,25.4 30.48,25.4 28.57,27.3 24.13,27.3 22.86,28.57 v22.86,29.21 | X1.4 40.01,27.05
  Top 0.406: IC2.1 65.91,32.51 v66.04,32.39
  Bottom 0.254: v43.81,31.12 48.26,31.12 50.16,33.02 58.42,33.02 59.05,32.39 v66.04,32.39 | FOR_NANO.A5 46.35,24.13 40.01,17.78 X1.4
I2C_SDA  (via drill 0.5, 0.9)
  Top 0.254: RN6.4 45.16,29.66 v44.45,28.96 | 40,28.33 v40.01,28.32 37.85,28.32 37.47,27.94 29.84,27.94 28.57,29.21 v25.4,29.21 | X1.3 42.55,17.78 41.27,19.05 v41.27,26.04
  Top 0.406: IC2.2 65.28,31.24 v66.04,30.48
  Bottom 0.254: 65.41,31.12 v66.04,30.48 50.8,30.48 48.26,27.94 45.47,27.94 v44.45,28.96 40.64,28.96 v40.01,28.32 41.27,27.05 v41.27,26.04 | FOR_NANO.A4 46.99,21.59 42.55,17.15 X1.3
N$1
  Top 0.813: H1.2 3.88,24.77 | D1.C 10.52,26.4 12.19,26.38 IC1.8 | CD1.2 3.83,24.15 4.45,24.77
  Top 1.016: 3.88,24.77 4.45,24.77 8.89,24.77 10.52,26.4
N$2
  Top 0.254: POWER.A 5.2,12.46 4.83,12.83 4.83,14.1 RNB.3
  Top 0.406: 4.95,14.14 RNB.3
N$3  (via drill 0.5)
  Top 0.813: IC1.1 12.04,19.03 v10.79,17.78 | v8.26,27.94 7.72,27.94 CD1.1
  Bottom 0.813: v10.79,17.78 10.79,25.4 v8.26,27.94
N$6  (via drill 0.5)
  Top 0.254: IC2.5 60.2,27.43 59.05,28.57 59.05,40 58.42,40.64 21.59,40.64 v20.95,40 | v17.14,40 15.88,40 15.24,40.64 15.24,42.55 14.61,43.18 12.57,43.18 12.19,42.8 12.19,41.4 11.94,41.15 11.41,41.15 RN1.2
  Top 0.406: RN1.2 8.36,41.17 7.62,41.91 7.62,43.56 U$18.B1
  Bottom 0.254: v20.95,40 v17.14,40
N$7  (via drill 0.5)
  Top 0.254: IC2.4 60.2,28.7 59.69,29.21 59.69,40.64 59.05,41.27 20.32,41.27 19.68,40.64 v19.68,38.73 | v17.14,38.1 12.7,38.1 12.19,38.61 12.19,40.13 11.94,40.39 11.41,40.39 RN1.3
  Top 0.406: RN1.3 8.27,40.37 U$18.B2
  Bottom 0.254: v19.68,38.73 19.05,38.1 v17.14,38.1
N$8
  Top 0.254: IC2.3 60.83,29.97 60.33,30.48 60.33,41.27 59.69,41.91 19.05,41.91 18.41,41.27 18.41,37.47 17.78,36.83 12.7,36.83 11.43,38.1 11.43,39.53 RN1.4
  Top 0.406: RN1.4 6.53,39.57 U$18.B3
N$20  (via drill 0.5)
  Top 0.305: R1.C 100.85,33.14 v100.97,33.02 | v100.97,24.13 100.33,24.77 94.11,24.77 93.6,24.26 91.66,24.26 RN2.1
  Bottom 0.305: v100.97,33.02 v100.97,24.13
N$21
  Top 0.305: RN5.7 69.32,24.24 69.85,24.77 71.97,24.77 IC2.12 73.73,24.83 74.93,26.04 76,26.04 IC3.6
N$22
  Top 0.305: RN5.6 70.12,23.13 70.48,23.5 71.97,23.5 IC2.11 73.73,23.56 74.93,24.77 76,24.77 IC3.7
N$23
  Top 0.254: 71.97,22.23 IC2.10
  Top 0.305: RN5.5 70.92,21.18 IC2.10 73.73,22.29 74.93,23.5 76,23.5 IC3.8
N$29  (via drill 0.5)
  Top 0.305: R2.C 106.56,33.14 v106.68,33.02 | v106.68,24.77 106.05,25.4 93.73,25.4 93.34,25.02 91.62,25.02 RN2.2
  Bottom 0.305: v106.68,33.02 v106.68,24.77
N$30  (via drill 0.5)
  Top 0.305: R3.C 112.28,33.14 v112.39,33.02 | v112.39,25.4 111.76,26.04 93.47,26.04 93.22,25.78 91.62,25.78 RN2.3
  Bottom 0.305: v112.39,33.02 v112.39,25.4
N$31  (via drill 0.5)
  Top 0.305: R4.C 118,33.14 v118.11,33.02 | v118.11,27.94 116.84,26.67 91.67,26.67 RN2.4
  Bottom 0.305: v118.11,33.02 v118.11,27.94
N$32
  Top 0.305: RN3.8 140.26,31.68 140.97,32.39 140.97,37.35 R8.C
N$81  (via drill 0.5)
  Top 0.305: R7.C 135.14,33.14 v135.25,33.02 | v135.25,30.48 134.62,31.12 92.71,31.12 92.46,30.86 91.62,30.86 RN3.7
  Bottom 0.305: v135.25,33.02 v135.25,30.48
N$82  (via drill 0.5)
  Top 0.305: R6.C 129.43,33.14 v129.54,33.02 | v129.54,29.84 128.91,30.48 93.09,30.48 92.58,29.97 91.71,29.97 RN3.6
  Bottom 0.305: v129.54,33.02 v129.54,29.84
N$83  (via drill 0.5)
  Top 0.305: R5.C 123.71,33.14 v123.83,33.02 | v123.83,29.21 123.19,29.84 93.34,29.84 92.71,29.21 91.67,29.21 RN3.5
  Bottom 0.305: v123.83,33.02 v123.83,29.21
N$89
  Top 0.305: RN5.8 68.52,25.34 69.22,26.04 71.97,26.04 IC2.13 73.73,26.1 74.93,27.3 76,27.3 IC3.5
N$93
  Top 0.305: RN4.6 66.44,21.36 67.31,22.23 67.31,26.67 69.22,28.57 71.97,28.57 IC2.15 73.73,28.64 74.93,29.84 76,29.84 IC3.3
N$94
  Top 0.305: RN4.8 64.84,22.3 66.04,23.5 66.04,27.94 69.22,31.12 71.94,31.12 IC2.17 73.76,31.21 74.93,32.39 76,32.39 IC3.1
N$203
  Bottom 2.54: X251.2 154.33,45.74 154.31,45.72 K8_B1.COM@2 K8_B1.COM@1
N$204
  Top 2.54: K8_B1.NC 151.76,57.79 149.22,60.33 149.22,63.45 X251.3
N$205
  Top 2.54: K8_B1.NO 156.84,57.79 159.38,60.33 159.38,63.45 X251.1
N$206
  Top 2.54: K7_B1.NO 141.6,57.79 144.15,60.33 144.15,63.45 X261.1
N$207
  Top 2.54: K6_B1.NO 126.36,57.79 128.91,60.33 128.91,63.45 X271.1
N$208
  Top 2.54: K7_B1.NC 136.53,57.79 133.99,60.33 133.99,63.45 X261.3
N$209
  Bottom 2.54: K7_B1.COM@2 139.06,45.72 | 139.06,45.72 K7_B1.COM@1 | X261.2 139.09,45.74 139.06,45.72
N$210
  Top 2.54: K6_B1.NC 121.28,57.79 118.75,60.33 118.75,63.45 X271.3
N$211
  Bottom 2.54: K6_B1.COM@2 123.83,45.72 | 123.83,45.72 K6_B1.COM@1 | X271.2 123.85,45.74 123.83,45.72
N$212
  Top 2.54: K5_B1.NC 106.05,57.79 103.5,60.33 103.5,63.45 X281.3
N$213
  Bottom 2.54: K5_B1.COM@2 108.58,45.72 | 108.58,45.72 K5_B1.COM@1 | X281.2 108.61,45.74 108.58,45.72
N$214
  Top 2.54: K5_B1.NO 111.12,57.79 113.67,60.33 113.67,63.45 X281.1
N$215
  Top 2.54: K4_B1.NO 72.39,57.79 74.93,60.33 74.93,63.45 X291.1
N$216
  Top 2.54: K4_B1.NC 67.31,57.79 64.77,60.33 64.77,63.45 X291.3
N$217
  Bottom 2.54: K4_B1.COM@2 69.85,45.72 | 69.85,45.72 K4_B1.COM@1 | X291.2 69.87,45.74 69.85,45.72
N$218
  Top 2.54: K3_B1.NO 57.15,57.79 59.69,60.33 59.69,63.45 X301.1
N$219
  Top 2.54: K3_B1.NC 52.07,57.79 49.53,60.33 49.53,63.45 X301.3
N$220
  Bottom 2.54: K3_B1.COM@2 54.61,45.72 | 54.61,45.72 K3_B1.COM@1 | X301.2 54.63,45.74 54.61,45.72
N$221
  Top 2.54: K2_B1.NO 41.91,57.79 44.45,60.33 44.45,63.45 X311.1
N$222
  Top 2.54: K2_B1.NC 36.83,57.79 34.29,60.33 34.29,63.45 X311.3
N$223
  Bottom 2.54: K2_B1.COM@2 39.37,45.72 | 39.37,45.72 K2_B1.COM@1 | X311.2 39.39,45.74 39.37,45.72
N$224
  Top 2.54: K1_B1.NO 26.67,57.79 29.21,60.33 29.21,63.45 X3211.1
N$225
  Top 2.54: K1_B1.NC 21.59,57.79 19.05,60.33 19.05,63.45 X3211.3
N$226
  Bottom 2.54: K1_B1.COM@2 24.13,45.72 | 24.13,45.72 K1_B1.COM@1 | X3211.2 24.15,45.74 24.13,45.72
OC_R1  (via drill 0.5)
  Top 0.305: RN2.8 89.95,24.26 88.77,24.26 88.14,23.62 IC3.11 85.8,23.5 v83.82,23.5 | v90.81,38.73 92.71,40.64 151.76,40.64 154.31,43.18 154.31,52.07 155.57,53.34 K8_B1.C1
  Bottom 0.305: v90.81,38.73 90.81,33.02 83.82,26.04 v83.82,23.5
OC_R2  (via drill 0.5)
  Top 0.305: RN2.7 89.99,25.02 88.39,25.02 88.27,24.89 IC3.12 85.8,24.77 v82.55,24.77 | v88.9,38.73 91.44,41.27 137.79,41.27 139.06,42.55 139.06,52.07 140.34,53.34 K7_B1.C1
  Bottom 0.305: v88.9,38.73 88.9,33.02 82.55,26.67 v82.55,24.77
OC_R3  (via drill 0.5)
  Top 0.305: RN2.6 89.99,25.78 88.52,25.78 88.14,26.16 IC3.13 81.53,26.16 81.41,26.04 v81.28,26.04 | v87,38.73 90.17,41.91 122.56,41.91 123.83,43.18 123.83,52.07 125.09,53.34 K6_B1.C1
  Bottom 0.305: v87,38.73 87,33.02 81.28,27.3 v81.28,26.04
OC_R4  (via drill 0.5)
  Top 0.305: RN2.5 89.94,26.67 88.9,26.67 88.14,27.43 IC3.14 85.8,27.3 v80.01,27.3 | v85.09,38.73 88.9,42.55 107.31,42.55 108.58,43.81 108.58,52.07 109.86,53.34 K5_B1.C1
  Bottom 0.305: v85.09,38.73 85.09,33.02 80.01,27.94 v80.01,27.3
OC_R5  (via drill 0.5)
  Top 0.305: RN3.4 89.94,29.21 88.9,29.21 88.39,28.7 IC3.15 85.8,28.83 79.63,28.83 v79.38,28.57 | v83.19,38.73 80.01,41.91 75.56,41.91 74.93,42.55 74.93,52.7 74.3,53.34 K4_B1.C1
  Bottom 0.305: v83.19,38.73 83.19,32.39 v79.38,28.57
OC_R6  (via drill 0.5)
  Top 0.305: RN3.3 89.9,29.97 IC3.16 85.8,30.1 79.63,30.1 79.38,29.84 v78.74,29.84 | v81.28,38.73 79.38,40.64 62.87,40.64 62.23,41.27 62.23,52.7 61.59,53.34 K3_B1.C1
  Bottom 0.305: v81.28,38.73 81.28,31.75 79.38,29.84 v78.74,29.84
OC_R7  (via drill 0.5)
  Top 0.305: RN3.2 89.99,30.86 88.52,30.86 88.14,31.24 IC3.17 85.8,31.12 v78.11,31.12 | v79.38,38.73 78.11,40 62.23,40 61.59,40.64 61.59,41.91 60.33,43.18 44.45,43.18 43.81,43.81 43.81,52.7 43.18,53.34 K2_B1.C1
  Bottom 0.305: v79.38,38.73 79.38,34.29 80.01,33.66 80.01,31.75 79.38,31.12 v78.11,31.12
OC_R8  (via drill 0.5)
  Top 0.305: RN3.1 89.95,31.62 88.9,31.62 88.01,32.51 IC3.18 84.2,32.51 84.07,32.39 v78.74,32.39 | v77.47,38.73 62.23,38.73 60.96,40 60.96,41.53 59.94,42.55 29.21,42.55 28.57,43.18 28.57,52.7 27.94,53.34 K1_B1.C1
  Bottom 0.305: v77.47,38.73 77.47,34.29 v78.74,32.39
REG_5V  (via drill 0.5, 0.9)
  Top 0.254: v60.33,26.04 59.82,26.04 59.69,26.16 | RN6.6 RN6.5 47.23,29.59 47.75,29.59 48.13,29.97 v48.51,29.97 | 62.74,26.16 IC2.6 | 70.36,32.51 IC2.18 73.15,32.51
  Top 0.305: R1.A 102.35,38.85 102.87,39.37 107.95,39.37 | 107.95,39.37 113.67,39.37 | 113.67,39.37 119.38,39.37 | 119.38,39.37 125.09,39.37 | 125.09,39.37 130.81,39.37 | 130.81,39.37 136.53,39.37 | 136.53,39.37 141.6,39.37 142.24,38.73 142.24,37.58 R8.A | R7.A 136.64,39.25 136.53,39.37 | R6.A 130.93,39.25 130.81,39.37 | R5.A 125.21,39.25 125.09,39.37 | R4.A 119.5,39.25 119.38,39.37 | R3.A 113.78,39.25 113.67,39.37 | R2.A 108.06,39.25 107.95,39.37 | H1.1 7.46,19.27 4.95,16.76 4.95,15.83 RNB.6
  Top 0.406: U$18.A3 U$18.A2 U$18.A1 | 70.36,32.51 69.85,33.02 69.85,36.47 CB3.2 CA3.2 65.38,34.9 v64.77,34.29 | v1.91,18.41 4.45,20.95 7.37,20.95 H1.1
  Top 0.61: 69.22,37.11 CB3.2 | FOR_NANO.5V 57.66,31.75 58.29,31.12 58.29,26.92 59.05,26.16 | v48.51,29.97 48.51,28.19 45.09,24.77 X1.2 | C1.+ 96.77,38.35
  Top 0.813: 73.15,32.51 73.66,33.02 73.66,33.66 74.3,34.29 88.9,34.29 93.34,38.73 97.16,38.73 | 97.16,38.73 102.23,38.73 102.35,38.85 | 96.77,38.35 97.16,38.73 | 59.05,26.16 59.69,26.16 62.74,26.16 | 16.13,20.83 9.96,20.83 H1.1 | 16.13,20.83 17.27,20.83 18.41,19.69 20.75,19.69 C4.1 | IC1.4 16.13,19.15 16.13,20.83
  Top 1.016: H1.1 9.27,18.41 9.27,17.65 9.4,17.53 9.4,5.59 13.46,1.52 37.72,1.52 38.73,2.54 38.73,6.35 39.37,6.99 44.83,6.99 v45.09,7.24 45.21,7.37 | 22.05,19.69 22.23,19.69 22.86,20.32 22.86,26.67 v20.32,29.21
  Top 1.27: 20.75,19.69 22.05,19.69
  Bottom 0.254: U$18.A3 3.17,25.4 1.91,24.13 v1.91,18.41
  Bottom 0.61: FOR_NANO.5V 50.29,31.75 v48.51,29.97
  Bottom 0.813: v60.33,26.04 67.31,26.04 68.58,27.3 68.58,33.02 67.31,34.29 v64.77,34.29
  Bottom 1.016: v45.09,7.24 X1.2
REG_12V  (via drill 0.5)
  Top 0.61: IC1.7 13.46,23.16 | 14.1,22.48 14.15,22.48
  Top 0.813: v18.41,22.48 14.15,22.48 13.46,23.16 | v25.4,22.48 26.04,21.84 C3.1 26.04,14.61 27.3,13.34 BRA1.+
  Bottom 0.813: v18.41,22.48 v25.4,22.48
UNREG_12V  (via drill 0.5, 0.9)
  Top 0.762: v95.38,22.35 IC3.10
  Top 2.54: X2.2 26.97,7.32 21.59,12.7 BRA1.~@1 21.59,15.24 | 21.59,15.24 BRA1.~@2 | U$1.TIP 15.14,13.87 16.51,15.24 21.59,15.24
  Bottom 1.016: K1_B1.C2 19.68,53.34 19.05,52.7 19.05,41.91 | K2_B1.C2 34.92,53.34 34.29,52.7 34.29,41.91 | K3_B1.C2 50.16,53.34 49.53,52.7 49.53,41.91 50.29,41.91 | K4_B1.C2 65.41,53.34 64.77,52.7 64.77,41.91 | 67.31,41.91 67.94,41.91 | K5_B1.C2 104.14,53.34 103.5,52.7 103.5,42.55 104.14,41.91 | 98.81,41.91 99.06,41.91 | K6_B1.C2 119.38,53.34 118.75,52.7 118.75,42.55 118.11,41.91 | 116.84,41.91 116.59,41.91 | K7_B1.C2 134.62,53.34 133.99,52.7 133.99,41.91 | 134.37,41.91 134.62,41.91 | K8_B1.C2 149.86,53.34 149.22,52.7 149.22,41.91
  Bottom 1.27: 98.81,41.91 98.81,25.78 v95.38,22.35 | C2.+ 6.35,48.9 7.62,47.62 8.89,47.62 9.53,46.99 9.53,43.81 10.16,43.18 17.78,43.18 19.05,41.91 | v27.94,31.75 27.94,41.91
  Bottom 1.676: 67.94,41.91 98.81,41.91 | 99.06,41.91 104.14,41.91 116.59,41.91 | 116.84,41.91 118.11,41.91 133.99,41.91 134.37,41.91 | 134.62,41.91 149.22,41.91
  Bottom 1.778: 49.53,41.91 34.29,41.91 27.94,41.91 19.05,41.91 | 67.31,41.91 64.77,41.91 50.29,41.91 | v27.94,31.75 27.94,5.44 X2.2

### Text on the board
tNames: NC | COM | NO | NC | COM | NO | NC | COM | NO | NC | COM | NO | NC | COM | NO | NC | COM | NO | NC | COM | NO | NC | COM | NO | 1 | 4 | 5 | 8 | Bank 1 | A0 | A1 | A2 | Address | SC | SCL | SDA | +5V | GND | 2016 ControlEverything.com | MCP23008 | ANSR8G5V1 | REV.A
